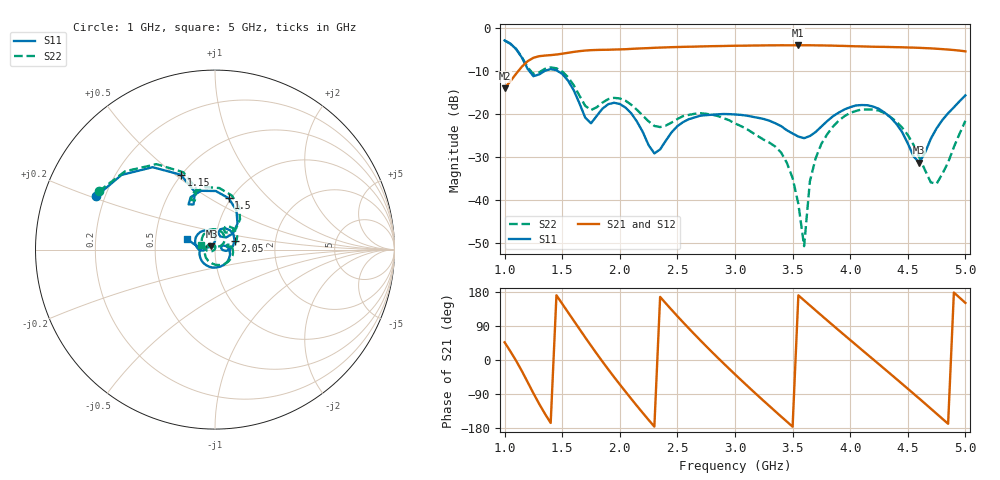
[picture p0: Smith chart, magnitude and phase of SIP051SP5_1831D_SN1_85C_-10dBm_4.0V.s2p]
# GHz  S  dB  R  50
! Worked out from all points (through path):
!   81 points, 1 GHz to 5 GHz, reference 50 ohm
!   highest |S21| = -3.89 dB at 3.55 GHz (marker M1); lowest = -13.9 dB at 1 GHz (marker M2)
!   lowest |S11| = -31.2 dB at 4.6 GHz (marker M3), VSWR 1.06, Z = 48 + j1.85 ohm
!   |S11| at or under -10 dB: 1.218 GHz to 1.341 GHz (122.9 MHz wide, 9.61 % of centre); 1.467 GHz to end of sweep
!   |S22| runs from -50.7 to -2.8 dB; largest |S21 - S12| = 0.0025
!   S11 on the Smith chart (normalised r, x): 1 GHz: 0.17, +0.21; 1.15 GHz: 0.50, +0.52; 1.5 GHz: 0.98, +0.61; 2.05 GHz: 1.24, +0.13; 5 GHz: 0.73, +0.09
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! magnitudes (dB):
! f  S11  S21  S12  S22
! 1 GHz  -2.8  -13.9  -13.9  -2.8
! 1.15 GHz  -6.8  -8.9  -8.9  -6.6
! 1.25 GHz  -11.1  -6.8  -6.8  -10.6
! 1.5 GHz  -10.6  -5.9  -5.9  -10.0
! 1.7 GHz  -20.8  -5.1  -5.1  -18.0
! 2.05 GHz  -18.4  -4.8  -4.8  -16.8
! 2.3 GHz  -29.1  -4.5  -4.5  -22.7
! 2.35 GHz  -28.2  -4.4  -4.4  -22.9
! 2.6 GHz  -21.1  -4.2  -4.2  -20.1
! 3 GHz  -20.0  -4.0  -4.0  -22.1
! 3.4 GHz  -22.7  -3.9  -3.9  -28.9
! 3.5 GHz  -24.4  -3.9  -3.9  -34.8
! 3.55 GHz  -25.2  -3.9  -3.9  -40.8
! 3.6 GHz  -25.5  -3.9  -3.9  -50.7
! 3.65 GHz  -25.0  -3.9  -3.9  -35.6
! 3.7 GHz  -24.1  -3.9  -3.9  -30.2
! 3.8 GHz  -21.6  -4.0  -4.0  -24.6
! 4 GHz  -18.3  -4.1  -4.1  -19.6
! 4.35 GHz  -20.7  -4.3  -4.3  -20.6
! 4.6 GHz  -31.2  -4.5  -4.5  -30.0
! 4.75 GHz  -23.2  -4.7  -4.7  -36.2
! 5 GHz  -15.6  -5.3  -5.3  -21.5
